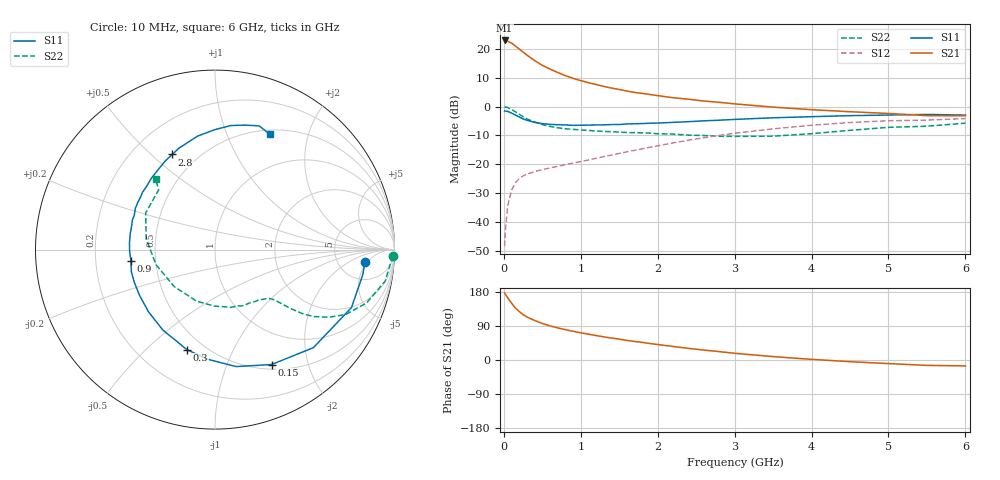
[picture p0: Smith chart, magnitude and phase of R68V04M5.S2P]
! SIEMENS Small Signal Semiconductors
! BFR193
! Si NPN RF Bipolar Junction Transistor in SOT23
! VCE = 8 V  IC = 4.5 mA
! Common Emitter S-Parameters:  May  1996
# GHz  S  MA  R  50
!  f  S11  S21  S12  S22
! GHz  MAG  ANG  MAG  ANG  MAG  ANG  MAG  ANG
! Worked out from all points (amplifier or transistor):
!   36 points, 10 MHz to 6 GHz, reference 50 ohm
!   highest |S21| = 22.9 dB at 10 MHz (marker M1)
!   |S21| within 3 dB of that: start of sweep to 201.3 MHz
!   unconditionally stable (mu >= 1): 954.6 MHz to 2.055 GHz
!   at 250 MHz: K = 0.40, MSG = 21.5 dB, |S12| = -24.1 dB
!   at 1.4 GHz: K = 1.06, MAG = 10.1 dB, |S12| = -16.8 dB
!   at 6 GHz: K = 0.96, MSG = 0.5 dB, |S12| = -4.1 dB
!   S11 on the Smith chart (normalised r, x): 10 MHz: 9, -4; 150 MHz: 0.56, -1.46; 300 MHz: 0.40, -0.68; 900 MHz: 0.36, -0.06; 2.8 GHz: 0.37, +0.58; 6 GHz: 0.55, +1.43
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0.01  0.8389 -4.8  14.03 176.9  0.0038 88.2  0.9916 -2.1
0.02  0.835 -9.7  13.95 173.3  0.0073 84.0  0.9814 -4.3
0.05  0.8262 -23.0  13.56 164.3  0.0189 77.9  0.9643 -10.5
0.1  0.7741 -44.9  12.66 150.0  0.0354 68.5  0.8953 -19.4
0.15  0.7136 -63.8  11.22 137.4  0.0477 60.0  0.813 -26.4
0.2  0.6622 -79.8  9.96 127.9  0.0565 54.6  0.738 -30.7
0.25  0.6122 -93.9  8.821 119.7  0.0627 50.7  0.6672 -34.0
0.3  0.5792 -105.6  7.82 113.4  0.0671 48.7  0.6127 -36.0
0.4  0.5341 -123.0  6.279 104.3  0.075 46.5  0.5395 -37.8
0.5  0.5072 -137.0  5.198 96.4  0.0806 46.3  0.4881 -38.9
0.6  0.4917 -148.9  4.473 90.1  0.0865 47.0  0.4526 -39.7
0.7  0.4852 -158.0  3.904 84.7  0.0921 48.6  0.4296 -40.5
0.9  0.4724 -172.5  3.088 75.8  0.1051 51.4  0.4029 -42.4
1.1  0.478 175.2  2.602 68.1  0.1188 54.5  0.3855 -45.8
1.3  0.4821 164.8  2.238 61.1  0.1359 56.9  0.3708 -49.4
1.6  0.4999 152.6  1.86 51.7  0.1644 58.9  0.3552 -56.4
2.2  0.533 131.6  1.425 35.6  0.2345 58.2  0.3338 -74.6
2.8  0.5811 114.2  1.187 22.1  0.3166 52.7  0.3059 -99.9
3.5  0.6395 98.8  0.979 9.0  0.4117 42.5  0.3069 -138.0
4.5  0.6969 82.7  0.815 -4.4  0.5297 25.5  0.3877 171.2
5.5  0.7318 70.4  0.697 -14.2  0.5829 7.9  0.4573 133.4
6  0.7126 64.7  0.693 -15.5  0.6202 2.9  0.516 129.9
